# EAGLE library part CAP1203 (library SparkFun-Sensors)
CAP1203 Sensor A 3 channel, I2C based capacitive touch sensor
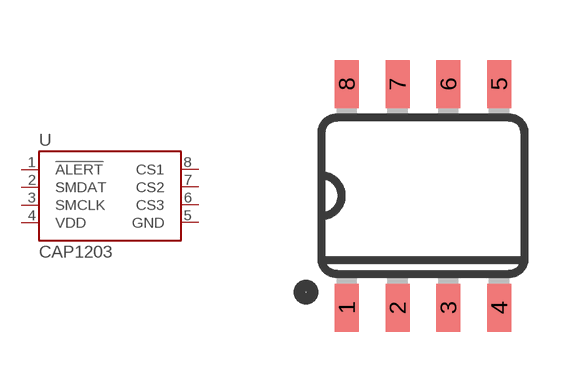
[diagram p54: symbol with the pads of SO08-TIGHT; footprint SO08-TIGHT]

Designator prefix U

## CAP1203 (PROD_ID: IC-14356; VALUE: CAP1203)  [SO08-TIGHT]
1  !ALERT  out
2  SMDAT
3  SMCLK  in
4  VDD  pwr
5  GND  pwr
6  CS3
7  CS2
8  CS1

## Footprint SO08-TIGHT (pad centres in mm)
smd 0.6 x 1.2: 1 -1.905,-2.8; 2 -0.635,-2.8; 3 0.635,-2.8; 4 1.905,-2.8; 5 1.905,2.8; 6 0.635,2.8; 7 -0.635,2.8; 8 -1.905,2.8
